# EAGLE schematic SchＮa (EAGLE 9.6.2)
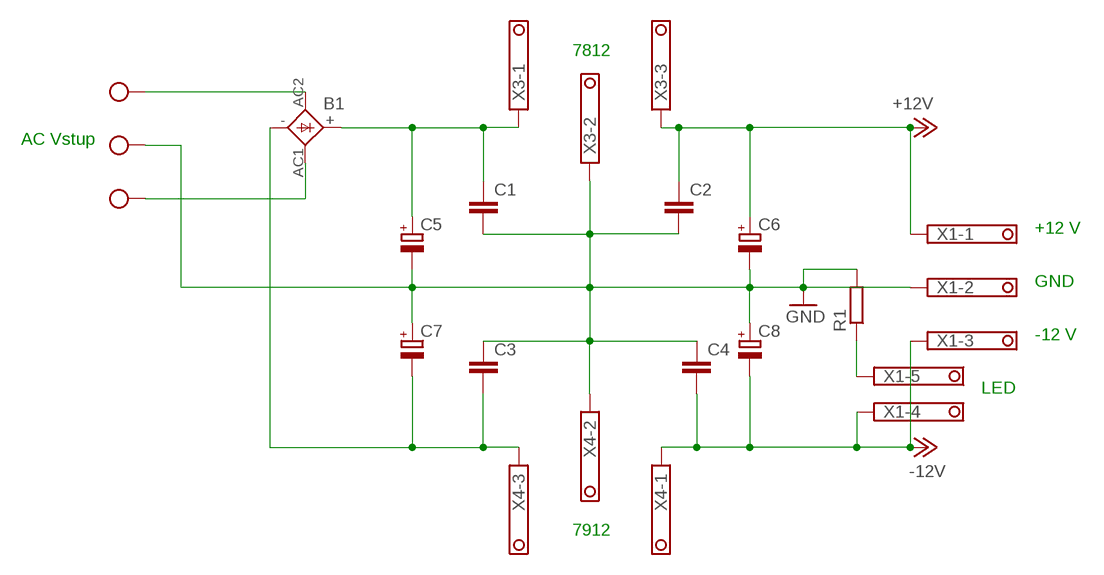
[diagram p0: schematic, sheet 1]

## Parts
B1  KBL  [KBL]
C1  C5/3.5  [C5B3.5]
C2  C5/3.5  [C5B3.5]
C3  C5/3.5  [C5B3.5]
C4  C5/3.5  [C5B3.5]
C5  CPOL-EUE5-13  [E5-13]
C6  CPOL-EUE5-6  [E5-6]
C7  CPOL-EUE5-13  [E5-13]
C8  CPOL-EUE5-6  [E5-6]
R1  R-EU_0207/10  [0207/10]
X1  1751277  [1751277]
X3  1751251  [1751251]
X4  1751251  [1751251]
X6  AK500/3  [AK500/3]

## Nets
+12V: C2.1 C6.+ X1.1 X3.3
-12V: C4.2 C8.- X1.3 X1.4 X4.1
GND: C1.2 C2.2 C3.1 C4.1 C5.- C6.- C7.+ C8.+ R1.2 X1.2 X3.2 X4.2 X6.2
N$1: R1.1 X1.5
N$2: B1.- C3.2 C7.- X4.3
N$3: B1.+ C1.1 C5.+ X3.1
N$4: B1.AC2(AC1) X6.3
N$5: B1.AC1(AC2) X6.1

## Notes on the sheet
- 7812
- AC Vstup
- +12 V
- GND
- -12 V
- LED
- 7912

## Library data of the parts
B1 = rectifier:KBL: DIOTEC RECTIFIER
C1-C4 = capacitor-wima:C: CAPACITOR
C5-C8 = rcl:CPOL-EU: POLARIZED CAPACITOR, European symbol; SPICEPREFIX: C
R1 = rcl:R-EU_: RESISTOR, European symbol; SPICEPREFIX: R
X1 = con-phoenix-350:1751277: MKDS 1/ 5-3,5 Printklemme Nennstrom: 10 A Bemessungsspannung: 160 V Raster: 3,5 mm Polzahl: 5 Montageart: Löten Anschlussart: Schraubanschluss Anschlussrichtung vom Leiter zur Platine: 0° Source: http://eshop.phoenixcontact.com .. 1751277.pdf; OC_FARNELL: unknown; OC_NEWARK: unknown
X3 X4 = con-phoenix-350:1751251: MKDS 1/ 3-3,5 Printklemme Nennstrom: 10 A Bemessungsspannung: 160 V Raster: 3,5 mm Polzahl: 3 Montageart: Löten Anschlussart: Schraubanschluss Anschlussrichtung vom Leiter zur Platine: 0° Source: http://eshop.phoenixcontact.com .. 1751251.pdf; OC_FARNELL: unknown; OC_NEWARK: unknown
X6 = con-ptr500:AK500/3: CONNECTOR; OC_FARNELL: unknown; OC_NEWARK: unknown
